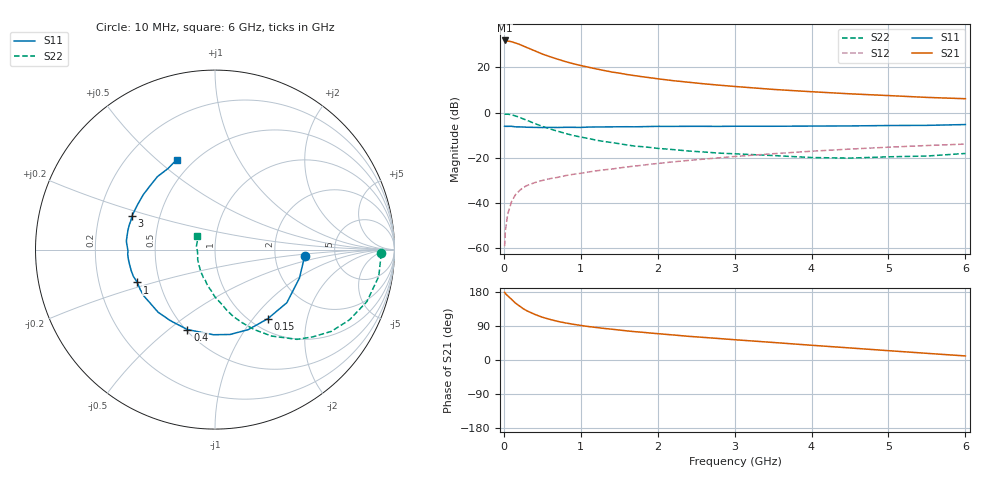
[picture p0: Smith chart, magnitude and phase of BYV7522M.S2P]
! SIEMENS Small Signal Semiconductors
! BFY420
! Si NPN RF SIEGET Grounded Emitter Transistor in MICRO-X
! VCE = 0.75 V  IC = 22 mA
! Common Emitter S-Parameters:  October  1996
# GHz  S  MA  R  50
!  f  S11  S21  S12  S22
! GHz  MAG  ANG  MAG  ANG  MAG  ANG  MAG  ANG
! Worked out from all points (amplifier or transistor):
!   36 points, 10 MHz to 6 GHz, reference 50 ohm
!   highest |S21| = 32.0 dB at 10 MHz (marker M1)
!   |S21| within 3 dB of that: start of sweep to 290.3 MHz
!   unconditionally stable (mu >= 1): start of sweep to 11.68 MHz; 1.597 GHz to end of sweep
!   at 250 MHz: K = 0.34, MSG = 31.4 dB, |S12| = -33.2 dB
!   at 1.4 GHz: K = 0.96, MSG = 21.5 dB, |S12| = -25.0 dB
!   at 6 GHz: K = 1.10, MAG = 8.1 dB, |S12| = -13.9 dB
!   S11 on the Smith chart (normalised r, x): 10 MHz: 2.97, -0.30; 150 MHz: 1.18, -1.19; 400 MHz: 0.51, -0.58; 1 GHz: 0.37, -0.18; 3 GHz: 0.35, +0.17; 6 GHz: 0.41, +0.58
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0.01  0.5007 -4.4  39.7 178.6  0.0011 97.4  0.924 -1.3
0.02  0.4966 -8.0  39.62 175.3  0.0024 90.5  0.9244 -3.2
0.05  0.4966 -18.6  38.52 169.4  0.0056 81.7  0.9245 -9.3
0.1  0.4978 -36.5  37.26 160.2  0.0106 77.4  0.8944 -18.9
0.15  0.4845 -52.7  34.96 150.3  0.0151 69.2  0.8452 -27.6
0.2  0.4829 -67.4  32.71 143.0  0.0185 65.7  0.7923 -35.1
0.25  0.4802 -80.0  30.07 135.6  0.0218 61.8  0.7289 -41.9
0.3  0.4744 -91.1  27.65 129.8  0.0242 60.2  0.6771 -47.6
0.4  0.4713 -109.0  23.47 120.6  0.0281 55.7  0.5757 -56.8
0.5  0.4675 -122.2  19.91 112.9  0.0314 53.3  0.4961 -63.9
0.6  0.4714 -132.3  17.32 107.1  0.0345 52.9  0.4357 -69.5
0.7  0.4683 -140.3  15.28 101.9  0.0368 51.9  0.3871 -74.6
0.8  0.4731 -146.8  13.52 97.9  0.0402 51.7  0.3462 -78.8
1  0.4701 -157.1  11.04 91.2  0.0453 52.8  0.2878 -85.7
1.1  0.4787 -161.9  10.14 88.3  0.0483 53.0  0.2665 -89.5
1.6  0.4869 -177.0  6.992 76.8  0.0625 53.3  0.1925 -104.4
2.2  0.496 170.9  5.109 66.1  0.0811 51.4  0.1519 -119.6
3  0.4992 157.7  3.799 53.5  0.1066 47.0  0.1224 -137.4
3.5  0.4988 149.7  3.271 46.3  0.1229 43.5  0.112 -149.4
4.5  0.5073 135.4  2.61 31.8  0.1557 34.3  0.0983 -173.1
5.5  0.5221 120.1  2.174 17.6  0.1868 24.2  0.1092 154.8
6  0.5442 113.2  2.033 10.7  0.201 19.0  0.1246 142.0
